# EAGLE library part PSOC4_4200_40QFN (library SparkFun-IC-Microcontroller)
Cypress PSoC 4200 32-bit MCU 48-MHz ARM Cortex-M0 Datasheet SparkFun Products: SparkFun serial Controlled Motor Driver
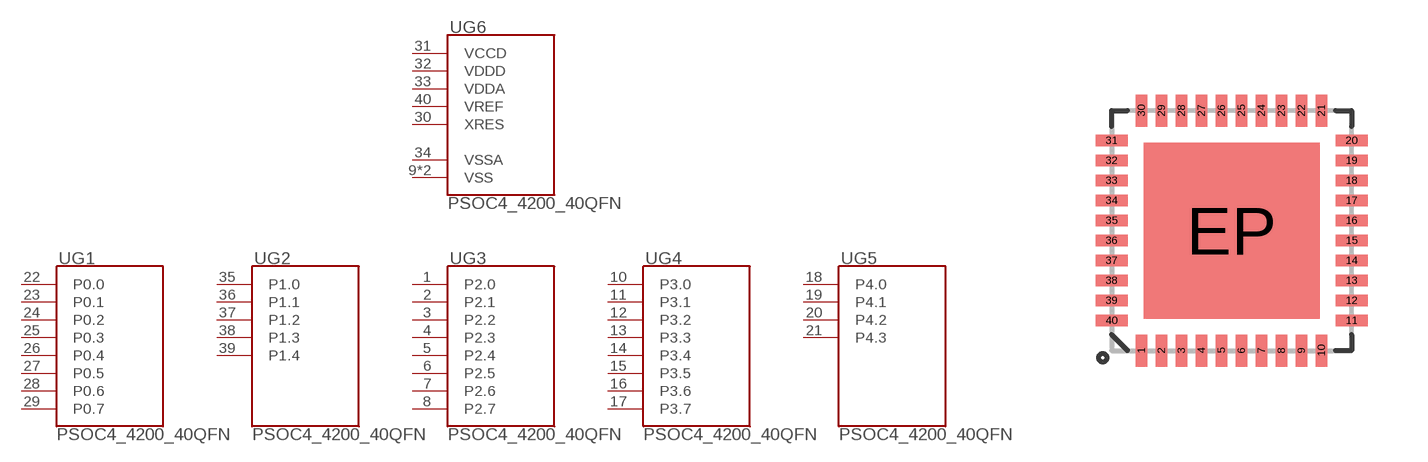
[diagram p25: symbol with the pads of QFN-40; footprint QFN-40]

Designator prefix U; gates G1=CY8C4245LQI_40QFN_PORT0 G2=CY8C4245LQI_40QFN_PORT1 G3=CY8C4245LQI_40QFN_PORT2 G4=CY8C4245LQI_40QFN_PORT3 G5=CY8C4245LQI_40QFN_PORT4 G6=CY8C4245LQI_40QFN_POWER

## PSOC4_4200_40QFN (PROD_ID: IC-13292; VALUE: CY8C4245LQI-483)  [QFN-40]
1  G3:P2.0
2  G3:P2.1
3  G3:P2.2
4  G3:P2.3
5  G3:P2.4
6  G3:P2.5
7  G3:P2.6
8  G3:P2.7
9  G6:VSS
10  G4:P3.0
11  G4:P3.1
12  G4:P3.2
13  G4:P3.3
14  G4:P3.4
15  G4:P3.5
16  G4:P3.6
17  G4:P3.7
18  G5:P4.0
19  G5:P4.1
20  G5:P4.2
21  G5:P4.3
22  G1:P0.0
23  G1:P0.1
24  G1:P0.2
25  G1:P0.3
26  G1:P0.4
27  G1:P0.5
28  G1:P0.6
29  G1:P0.7
30  G6:XRES
31  G6:VCCD
32  G6:VDDD
33  G6:VDDA
34  G6:VSSA
35  G2:P1.0
36  G2:P1.1
37  G2:P1.2
38  G2:P1.3
39  G2:P1.4
40  G6:VREF
EP  G6:VSS

## Footprint QFN-40 (pad centres in mm)
40-QFN from Cypress 4245 datasheet, with Sparkfun DFM
smd 0.285 x 0.8: 1 -2.25,-3; 2 -1.75,-3; 3 -1.25,-3; 4 -0.75,-3; 5 -0.25,-3; 6 0.25,-3; 7 0.75,-3; 8 1.25,-3; 9 1.75,-3; 10 2.25,-3; 21 2.25,3; 22 1.75,3; 23 1.25,3; 24 0.75,3; 25 0.25,3; 26 -0.25,3; 27 -0.75,3; 28 -1.25,3; 29 -1.75,3; 30 -2.25,3
smd 0.8 x 0.285: 11 3,-2.25; 12 3,-1.75; 13 3,-1.25; 14 3,-0.75; 15 3,-0.25; 16 3,0.25; 17 3,0.75; 18 3,1.25; 19 3,1.75; 20 3,2.25; 31 -3,2.25; 32 -3,1.75; 33 -3,1.25; 34 -3,0.75; 35 -3,0.25; 36 -3,-0.25; 37 -3,-0.75; 38 -3,-1.25; 39 -3,-1.75; 40 -3,-2.25
smd 4.4 x 4.4: EP 0,0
